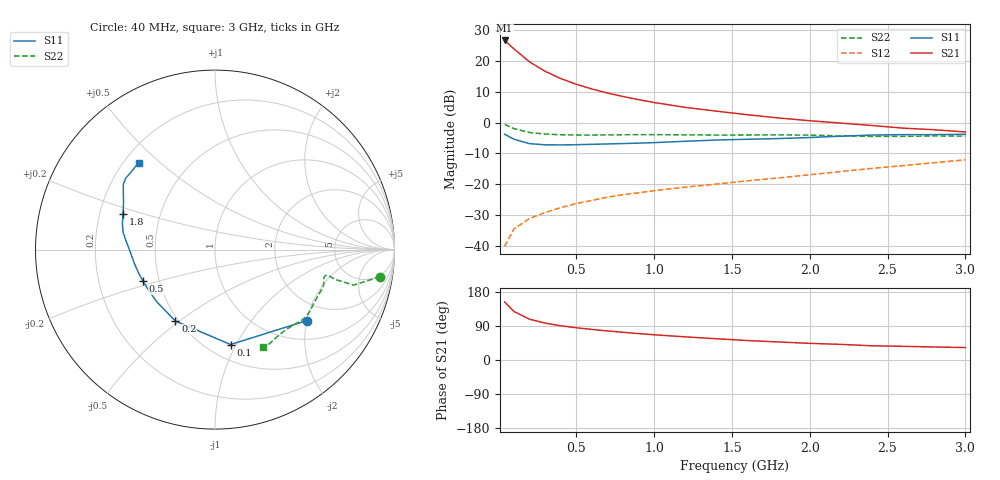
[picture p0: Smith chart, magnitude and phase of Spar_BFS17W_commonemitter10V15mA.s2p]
! Filename:  BFS17WI.S2P  Version:  4.0
! NXP part #: BFS17W  Date: Jun 1994
! Bias condition: Vce=10V, Ic=15mA
#  MHz  S  MA  R  50
! Freq  S11  S21  S12  S22  !GUM [dB]
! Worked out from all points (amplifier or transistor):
!   21 points, 40 MHz to 3 GHz, reference 50 ohm
!   highest |S21| = 26.5 dB at 40 MHz (marker M1)
!   |S21| within 3 dB of that: start of sweep to 106.6 MHz
!   unconditionally stable (mu >= 1): 366.3 MHz to 2.276 GHz
!   at 300 MHz: K = 0.93, MSG = 22.8 dB, |S12| = -29.1 dB
!   at 1 GHz: K = 1.19, MAG = 11.6 dB, |S12| = -22.0 dB
!   at 3 GHz: K = 0.93, MSG = 4.5 dB, |S12| = -12.1 dB
!   S11 on the Smith chart (normalised r, x): 40 MHz: 1.47, -2.00; 100 MHz: 0.64, -0.95; 200 MHz: 0.48, -0.48; 500 MHz: 0.41, -0.18; 1.8 GHz: 0.30, +0.17; 3 GHz: 0.26, +0.43
40  0.646 -37.8  21.24 153.1  0.01 73.2  0.933 -9.3
100  0.536 -80.7  15.53 127.9  0.019 60.6  0.797 -14.4
200  0.455 -119.0  9.578 107.6  0.028 58.0  0.689 -13.9
300  0.436 -138.0  6.734 97.3  0.035 59.5  0.651 -13.0
400  0.434 -149.2  5.154 90.3  0.042 62.3  0.634 -13.0
500  0.438 -156.4  4.161 85.1  0.049 63.7  0.628 -13.7
600  0.444 -162.1  3.49 80.7  0.055 65.5  0.627 -14.8
700  0.45 -166.8  3.003 76.8  0.062 67.1  0.63 -15.9
800  0.457 -171.0  2.637 73.1  0.068 68.2  0.634 -17.1
900  0.464 -175.0  2.343 69.7  0.073 69.3  0.636 -18.2
1000  0.473 -178.7  2.108 66.6  0.079 70.8  0.637 -19.5
1200  0.497 174.7  1.76 61.1  0.09 73.6  0.631 -22.5
1400  0.521 169.3  1.527 56.1  0.101 76.7  0.627 -26.6
1600  0.536 164.3  1.336 51.3  0.114 79.5  0.628 -31.1
1800  0.55 158.7  1.185 47.6  0.127 82.7  0.631 -35.0
2000  0.572 153.0  1.069 43.9  0.143 85.4  0.625 -38.6
2200  0.601 148.2  0.978 41.2  0.161 87.4  0.609 -43.1
2400  0.627 144.5  0.895 37.5  0.181 89.0  0.595 -49.0
2600  0.637 141.3  0.811 36.1  0.201 89.7  0.597 -55.1
2800  0.637 136.8  0.764 34.3  0.224 90.3  0.606 -60.0
3000  0.645 131.3  0.703 32.9  0.249 90.6  0.604 -63.8
